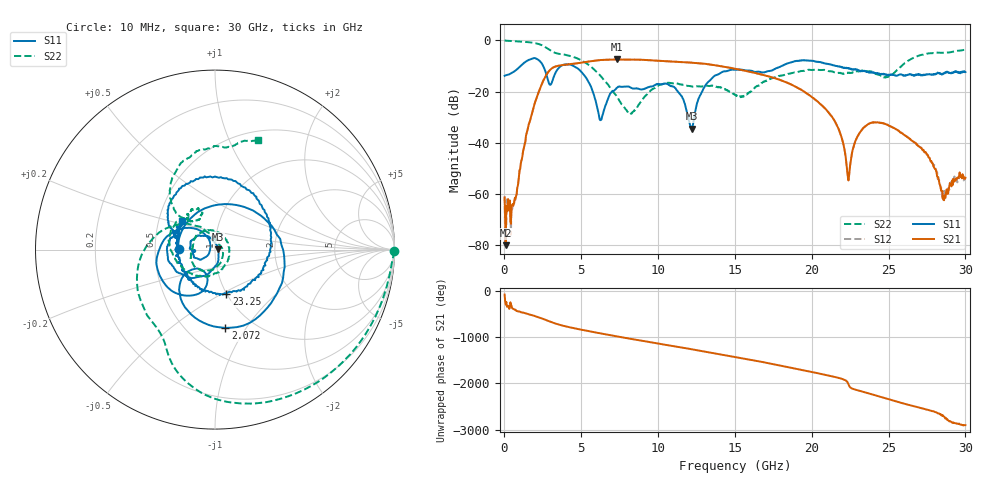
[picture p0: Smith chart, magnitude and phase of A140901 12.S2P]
!  2-Port S-parameters saved by WinCal
! VAR MeasName=S-Parameters (CALIBRATED_DATA) read from VNA (N5244A)
! VAR MeasDate=11/3/2014 9:27:41 AM
! VAR NAME=A140901 12
! VAR FILENAME=A140901 12.S2P
! VAR DATE=11/3/2014 9:27:41 AM
! VAR PHYS_PORTS=1,2
# Hz S RI R 50
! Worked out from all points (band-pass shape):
!   801 points, 10 MHz to 30 GHz, reference 50 ohm
!   highest |S21| = -7.47 dB at 7.32 GHz (marker M1); lowest = -80.3 dB at 84.97 MHz (marker M2)
!   |S21| within 3 dB of the highest: 3.215 GHz to 14.44 GHz (11.22 GHz wide, 127 % of centre)
!   lowest |S11| = -34.6 dB at 12.19 GHz (marker M3), VSWR 1.04, Z = 51.9 + j0.074 ohm
!   |S11| at or under -10 dB: 2.52 GHz to 3.683 GHz (1.164 GHz wide, 37.5 % of centre); 4.491 GHz to 18.05 GHz (13.56 GHz wide, 120 % of centre); 21.65 GHz to end of sweep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
!   |S22| runs from -28.9 to 0.0 dB; largest |S21 - S12| = 0.0036
!   S11 on the Smith chart (normalised r, x): 10 MHz: 0.66, +0.01; 2.072 GHz: 0.75, -0.81; 23.25 GHz: 1.00, -0.53; 30 GHz: 0.66, +0.22
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1e7  -0.2029 0.00448  0.000109 -0.000828  0.000555 0.000713  0.9984 -0.00873
8.4975e7  -0.2033 0.0426  4.79e-05 8.43e-05  -0.000161 0.000265  0.9873 -0.0622
5.723125e8  -0.0365 0.2368  0.000493 -0.000315  0.000488 -0.000265  0.9035 -0.3513
1.434525e9  0.3869 -0.0643  -0.0101 -0.011  -0.01 -0.0109  0.56 -0.7457
2.071812e9  0.0568 -0.4362  -0.0687 0.0222  -0.0687 0.0224  0.1701 -0.8576
3.533825e9  -0.1337 -0.2561  0.3158 -0.0591  0.3155 -0.0587  -0.3167 -0.4472
5.033325e9  -0.2116 0.1078  -0.2027 -0.3075  -0.2025 -0.3072  -0.4038 -0.0205
6.270412e9  -0.0276 0.000981  -0.3815 0.1599  -0.3814 0.159  -0.1419 0.1408
7.320062e9  -0.1079 -0.0475  -0.0235 0.4227  -0.024 0.4224  -0.0177 0.0783
8.219762e9  -0.1188 -0.0119  0.3192 0.2772  0.3191 0.2762  0.0303 0.0204
1.001916e10  -0.1409 0.0084  0.189 -0.3552  0.1878 -0.3547  -0.0542 -0.1201
1.219344e10  0.0187 0.000713  -0.3658 0.0268  -0.3657 0.0262  -0.1262 0.00289
1.316811e10  -0.041 -0.1375  -0.1657 0.3017  -0.1662 0.3023  -0.12 0.0486
1.5005e10  -0.2636 -0.0345  0.2745 0.0506  0.2747 0.0488  0.0545 0.0668
2.002832e10  0.0926 0.3901  0.0555 0.0534  0.0551 0.0538  -0.2498 0.0827
2.16028e10  0.312 0.0441  0.00783 -0.0214  0.00806 -0.0215  -0.1542 0.1704
2.239004e10  0.2417 -0.1414  -0.00127 0.00129  -0.00138 0.00132  -0.1569 0.1711
2.325225e10  0.064 -0.2459  0.017 -0.00445  0.0173 -0.00438  -0.1307 0.2194
2.501416e10  -0.1635 -0.1262  -0.0214 0.00136  -0.0214 0.0013  -0.1158 0.162
2.741336e10  -0.2107 0.0282  0.00501 -0.00422  0.00484 -0.00407  -0.131 0.5248
2.857548e10  -0.202 0.0982  -0.000743 0.000148  -0.000859 4.57e-05  0.0686 0.5705
3e10  -0.1818 0.1577  0.00188 -0.000777  0.00208 -0.000609  0.2417 0.6119
